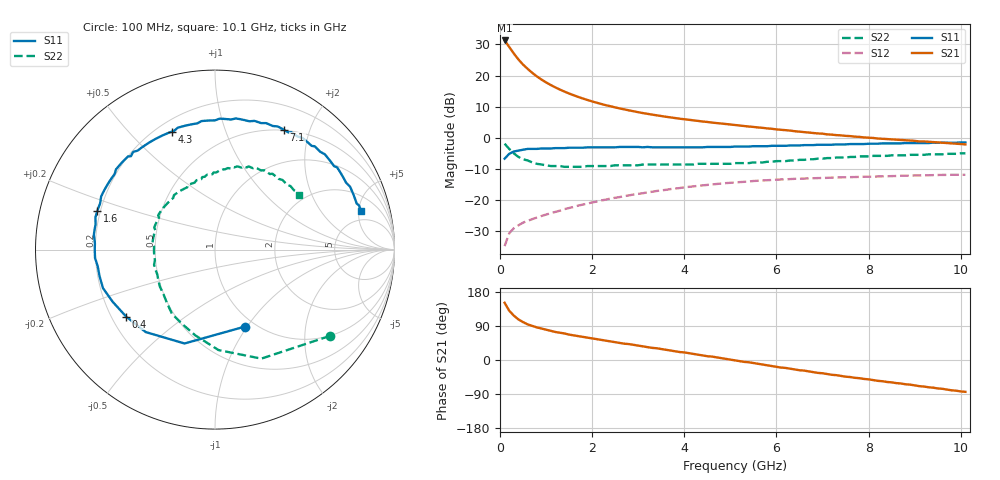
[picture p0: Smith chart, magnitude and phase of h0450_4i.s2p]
!HBFP-0450
!S and NOISE PARAMETERS at Vce=4V  Ic=70mA.  LAST UPDATED  09-04-98
# GHZ S MA R  50
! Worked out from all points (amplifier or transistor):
!   101 points, 100 MHz to 10.1 GHz, reference 50 ohm
!   highest |S21| = 31.3 dB at 100 MHz (marker M1)
!   |S21| within 3 dB of that: start of sweep to 243.2 MHz
!   unconditionally stable (mu >= 1): 2.201 GHz to end of sweep
!   at 1.7 GHz: K = 0.95, MSG = 17.5 dB, |S12| = -21.8 dB
!   at 5.1 GHz: K = 1.08, MAG = 7.6 dB, |S12| = -14.4 dB
!   at 10.1 GHz: K = 1.06, MAG = 3.5 dB, |S12| = -11.9 dB
!   lowest NFmin = 2.04 dB at 1.8 GHz
!   S11 on the Smith chart (normalised r, x): 100 MHz: 0.89, -0.97; 400 MHz: 0.26, -0.31; 1.6 GHz: 0.19, +0.15; 4.3 GHz: 0.26, +0.67; 7.1 GHz: 0.49, +1.62; 10.1 GHz: 3.55, +5.25
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0.1  0.46 -69.0  36.63 151.0  0.018 60.0  0.8 -37.0
0.2  0.55 -108.0  28.83 130.0  0.029 50.0  0.66 -67.0
0.3  0.6 -130.0  22.56 117.0  0.035 44.0  0.56 -88.0
0.4  0.62 -143.0  18.13 107.0  0.039 41.0  0.49 -103.0
0.5  0.64 -153.0  14.99 100.0  0.043 40.0  0.45 -115.0
0.6  0.66 -161.0  12.8 94.0  0.046 40.0  0.43 -124.0
0.7  0.66 -167.0  11.04 90.0  0.049 40.0  0.4 -132.0
0.8  0.66 -172.0  9.68 86.0  0.052 40.0  0.38 -139.0
0.9  0.67 -176.0  8.61 83.0  0.055 41.0  0.37 -146.0
1.1  0.67 177.0  7.04 77.0  0.061 41.0  0.35 -157.0
1.3  0.68 170.0  5.94 72.0  0.067 42.0  0.35 -166.0
1.6  0.69 162.0  4.81 65.0  0.077 41.0  0.34 -177.0
1.8  0.69 158.0  4.26 61.0  0.084 40.0  0.34 177.0
2.2  0.7 149.0  3.48 53.0  0.098 38.0  0.35 167.0
2.6  0.71 141.0  2.95 45.0  0.111 35.0  0.36 158.0
3.5  0.7 125.0  2.23 29.0  0.142 25.0  0.37 141.0
4.3  0.7 110.0  1.86 14.0  0.168 15.0  0.38 127.0
5.1  0.72 96.0  1.6 -1.0  0.19 4.0  0.39 113.0
6.8  0.76 65.0  1.19 -32.0  0.223 -21.0  0.45 83.0
7.1  0.77 60.0  1.13 -37.0  0.226 -25.0  0.47 78.0
8.5  0.81 38.0  0.94 -59.0  0.241 -44.0  0.52 58.0
10.1  0.84 15.0  0.78 -84.0  0.253 -67.0  0.56 33.0
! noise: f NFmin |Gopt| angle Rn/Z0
1.8  2.04  0.64  -149  0.12
2  2.07  0.64  -147  0.14
2.5  2.22  0.64  -137  0.22
3.5  2.5  0.67  -120  0.43
4  2.66  0.68  -110  0.63
5  2.95  0.71  -92  1.09
5.5  3.09  0.73  -82  1.48
7  3.53  0.76  -56  2.88
8  3.83  0.8  -40  4.12
10  4.41  0.83  -12  6.41
